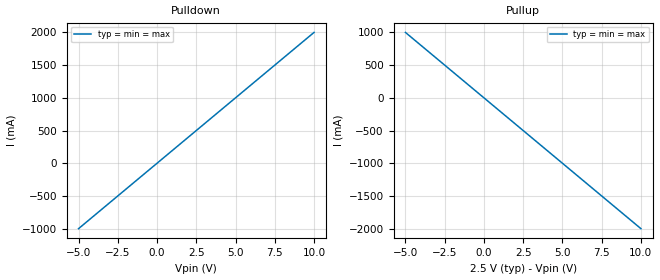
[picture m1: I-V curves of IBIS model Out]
[IBIS Ver]   3.2
[Comment Char]  |_char
[File Name]   bug41.ibs
[File Rev]   1.0
[Date]   May 9, 2000
[Component]   Test
[Manufacturer]   Test File
[Package]
| variable   typ   min   max
R_pkg   0.0m   NA   NA
L_pkg   0.0nH   NA   NA
C_pkg   0.0pF   NA   NA
[Pin]   signal_name   model_name   R_pin   L_pin   C_pin
  1   PAD   In   NA   NA   NA
  2   PAD   In   NA   NA   NA
  3   VTT   POWER   NA   NA   NA
  4   PADN   In   NA   NA   NA
[Series Pin Mapping]  pin_2   model_name   function_table_group
   1   2   Rseries
   2   3   Rseries
[Diff Pin]  inv_pin  vdiff  tdelay_typ tdelay_min tdelay_max
 1   3   150mV   -0ns   NA   NA
 2   3   150mV   0ns   NA   NA
 3   4   150mV   0ns   NA   NA
|   MODEL Rseries
[Model]   Rseries
Model_type   Series
C_comp   0.02pF   0.01pF  0.03pF
[Voltage Range]   2.50   2.30   2.70
| variable   R(typ)   R(min)   R(max)
[R Series]   100ohm   90ohm   110ohm
|   MODEL Term
[Model]   Term
Model_type   Terminator
Vinl  = 1.25V
Vinh = 2.5
C_comp   0.02pF   0.01pF  0.03pF
[Voltage Range]   2.50   2.30   2.70
|   MODEL In
[Model]   In
Model_type   Input
Vinl  = 1.25V
Vinh = 2.5
C_comp   0.02pF   0.01pF  0.03pF
[Voltage Range]   2.50   2.30   2.70
| Models and submodels in the file (4): Rseries (Series), Term (Terminator), In (Input), Out (Output)
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|   MODEL Out
[Model]   Out
Model_type   Output
Vmeas  = 1.25V
C_comp   0.02pF   0.01pF  0.03pF
[Voltage Range]   2.50   2.30   2.70
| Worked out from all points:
|   slope of the pulldown table from 0 to 0.375 V, typ, clamps not added: 5 ohm
|   slope of the pullup table from 0 to 0.375 V, typ, clamps not added: 5 ohm
[Pulldown]
-5V       -1A        -1A        -1A
10V       2A         2A         2A
[Pullup]
-5V       1A         1A         1A
10V       -2A        -2A        -2A
[Ramp]
dV/dt_r  1/1n 1/1n 1/1n
dV/dt_f  1/1n 1/1n 1/1n
